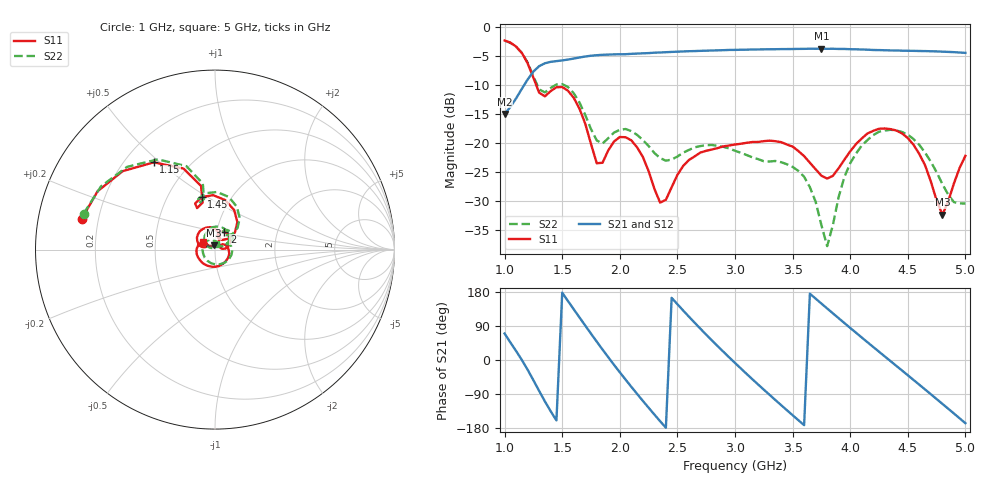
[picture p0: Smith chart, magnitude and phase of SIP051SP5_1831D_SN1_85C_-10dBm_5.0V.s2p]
# GHz  S  dB  R  50
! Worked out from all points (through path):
!   81 points, 1 GHz to 5 GHz, reference 50 ohm
!   highest |S21| = -3.78 dB at 3.75 GHz (marker M1); lowest = -15.0 dB at 1 GHz (marker M2)
!   lowest |S11| = -32.3 dB at 4.8 GHz (marker M3), VSWR 1.05, Z = 49.2 + j2.25 ohm
!   |S11| at or under -10 dB: 1.274 GHz to end of sweep
!   |S22| runs from -37.7 to -2.4 dB; largest |S21 - S12| = 0.0023
!   S11 on the Smith chart (normalised r, x): 1 GHz: 0.14, +0.11; 1.15 GHz: 0.32, +0.48; 1.45 GHz: 0.73, +0.47; 2 GHz: 1.09, +0.22; 5 GHz: 0.87, +0.07
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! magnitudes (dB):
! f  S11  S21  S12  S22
! 1 GHz  -2.4  -15.0  -15.0  -2.4
! 1.15 GHz  -4.5  -10.7  -10.6  -4.5
! 1.3 GHz  -11.3  -6.8  -6.8  -10.8
! 1.45 GHz  -10.4  -5.9  -5.9  -9.9
! 1.6 GHz  -12.2  -5.5  -5.5  -11.4
! 1.7 GHz  -16.7  -5.1  -5.1  -15.2
! 1.8 GHz  -23.5  -4.9  -4.9  -19.5
! 2 GHz  -19.0  -4.7  -4.7  -17.7
! 2.15 GHz  -20.7  -4.6  -4.6  -18.6
! 2.35 GHz  -30.2  -4.4  -4.4  -22.6
! 2.6 GHz  -22.9  -4.2  -4.2  -21.2
! 3 GHz  -20.3  -4.0  -4.0  -21.3
! 3.5 GHz  -20.6  -3.8  -3.8  -24.1
! 3.7 GHz  -24.5  -3.8  -3.8  -30.1
! 3.75 GHz  -25.6  -3.8  -3.8  -34.1
! 3.8 GHz  -26.1  -3.8  -3.8  -37.7
! 4 GHz  -21.4  -3.9  -3.9  -23.5
! 4.2 GHz  -17.9  -4.0  -4.0  -18.6
! 4.35 GHz  -17.6  -4.1  -4.1  -17.7
! 4.6 GHz  -21.9  -4.2  -4.2  -20.3
! 4.8 GHz  -32.3  -4.3  -4.3  -27.0
! 5 GHz  -22.2  -4.5  -4.5  -30.4
